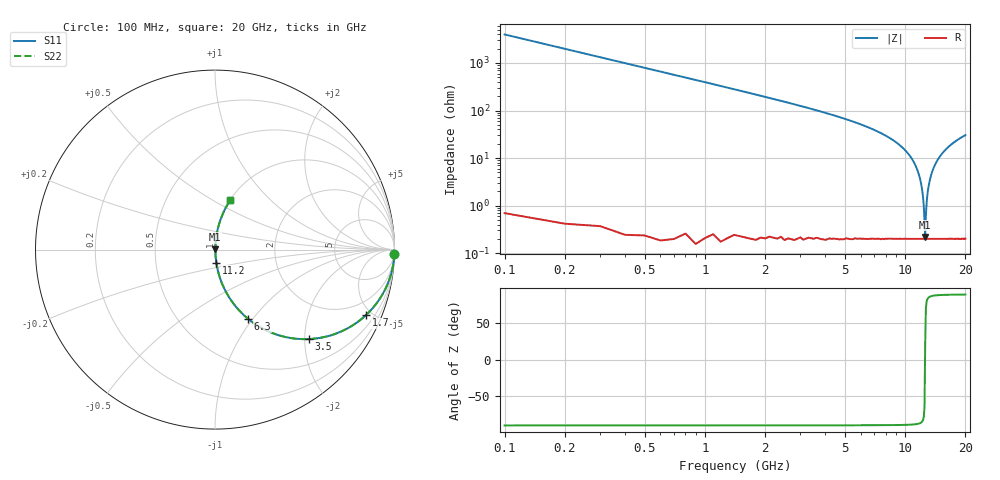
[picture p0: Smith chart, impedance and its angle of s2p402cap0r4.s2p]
! AVX Thin Film Operation		Date: April 2003
! Description: Accu-P® Series, Thin Film, SMD, RF Capacitor
! Part Number: 04021J0R4ABS
! 50 MHz  -  20 GHz
! Serial Measurements
# hz S db R 50
!	S11		S21		S12		S22
!	dB	Phase	dB	Phase	dB	Phase	dB	Phase
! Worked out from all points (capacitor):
!   200 points, 100 MHz to 20 GHz, reference 50 ohm
!   read as one part in series: C = 400 fF near 200 MHz
!   lowest |Z| = 219 mohm at 12.6 GHz (marker M1)
!   series resonance near 12.58 GHz, so ESL is about 400 pH
!   S11 on the Smith chart (normalised r, x): 100 MHz: 1, -80; 1.7 GHz: 1.00, -4.60; 3.5 GHz: 1.00, -2.10; 6.3 GHz: 1.00, -0.95; 11.2 GHz: 1.00, -0.15; 20 GHz: 1.00, +0.61
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1e8  -0.00 -1.4  -32.00 88.5  -32.00 88.5  -0.00 -1.4
2e8  -0.01 -2.9  -25.98 87.1  -25.98 87.1  -0.01 -2.9
3e8  -0.02 -4.3  -22.47 85.7  -22.47 85.7  -0.02 -4.3
6e8  -0.10 -8.6  -16.51 81.4  -16.51 81.4  -0.10 -8.6
1.1e9  -0.33 -15.6  -11.43 74.4  -11.43 74.4  -0.33 -15.6
1.7e9  -0.76 -23.5  -7.98 66.4  -7.98 66.4  -0.76 -23.5
3.5e9  -2.82 -43.6  -3.23 46.3  -3.23 46.3  -2.82 -43.6
6.3e9  -7.39 -64.5  -0.89 25.3  -0.89 25.3  -7.39 -64.5
6.8e9  -8.36 -67.3  -0.70 22.5  -0.70 22.5  -8.36 -67.3
1.01e10  -17.17 -81.2  -0.10 8.0  -0.10 8.0  -17.17 -81.2
1.12e10  -22.68 -84.2  -0.04 4.2  -0.04 4.2  -22.68 -84.2
1.18e10  -27.84 -84.9  -0.02 2.3  -0.02 2.3  -27.84 -84.9
1.22e10  -34.17 -83.0  -0.02 1.1  -0.02 1.1  -34.17 -83.0
1.24e10  -40.51 -77.2  -0.02 0.5  -0.02 0.5  -40.51 -77.2
1.26e10  -53.21 23.9  -0.02 -0.1  -0.02 -0.1  -53.21 23.9
1.27e10  -44.14 70.9  -0.02 -0.3  -0.02 -0.3  -44.14 70.9
1.29e10  -35.99 81.9  -0.02 -0.9  -0.02 -0.9  -35.99 81.9
1.31e10  -31.86 84.1  -0.02 -1.5  -0.02 -1.5  -31.86 84.1
1.34e10  -28.01 84.8  -0.02 -2.3  -0.02 -2.3  -28.01 84.8
1.46e10  -20.55 83.4  -0.06 -5.4  -0.06 -5.4  -20.55 83.4
1.67e10  -14.98 79.1  -0.16 -10.3  -0.16 -10.3  -14.98 79.1
2e10  -10.75 72.8  -0.40 -16.9  -0.40 -16.9  -10.75 72.8
